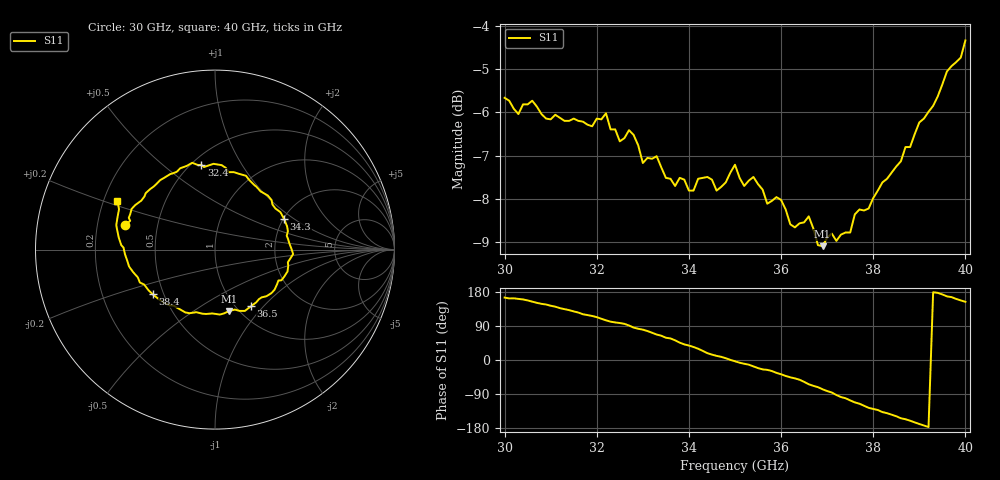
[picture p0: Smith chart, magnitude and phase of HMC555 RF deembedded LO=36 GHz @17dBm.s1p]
!Hittite Microwave Corporation
!20 Alpha Road
!Chelmsford, MA 01824
!Tel: 978-250-3343
!Fax: 978-250-3373
!Device: HMC555, 32-38GHz, I/Q Mixer
!Misc: RF Return Loss with LO = 36 GHz @ 17 dBm, Data includes one K connector, Room
# MHZ S MA R 50
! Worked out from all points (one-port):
!   101 points, 30 GHz to 40 GHz, reference 50 ohm
!   lowest |S11| = -9.1 dB at 36.9 GHz (marker M1), VSWR 2.08, Z = 45.3 - j35.4 ohm
!   |S11| at or under -10 dB: nowhere
!   S11 on the Smith chart (normalised r, x): 30 GHz: 0.32, +0.12; 32.4 GHz: 0.56, +0.68; 34.3 GHz: 2.02, +0.84; 36.5 GHz: 1.16, -0.85; 38.4 GHz: 0.44, -0.27; 40 GHz: 0.26, +0.22
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30000  0.521 164.7
30300  0.499 161.2
30600  0.517 154.0
31300  0.49 134.2
32000  0.493 113.1
32200  0.5 104.7
32400  0.479 99.2
32500  0.464 97.6
32700  0.478 91.0
33000  0.438 80.1
33300  0.446 67.2
33800  0.421 45.8
34300  0.421 24.0
34600  0.407 10.9
35000  0.436 -3.3
35600  0.408 -24.8
36300  0.369 -48.5
36500  0.374 -57.7
36600  0.38 -64.0
36900  0.351 -77.2
37500  0.364 -106.6
37700  0.387 -115.3
38400  0.427 -144.3
38800  0.457 -160.2
39000  0.488 -168.9
39400  0.523 177.2
39600  0.559 167.9
40000  0.607 153.6
